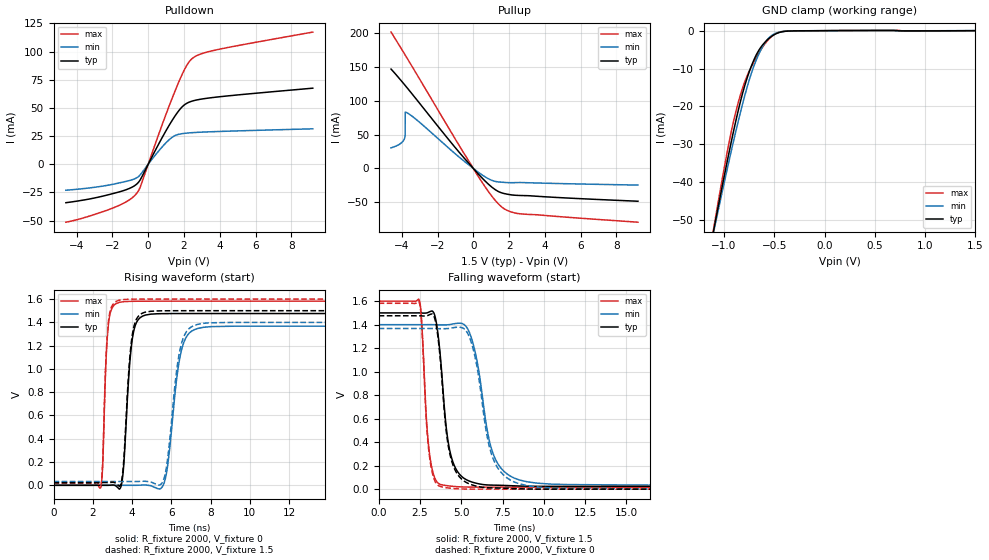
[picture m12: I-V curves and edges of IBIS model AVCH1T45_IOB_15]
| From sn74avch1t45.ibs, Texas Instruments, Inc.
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[Model]   AVCH1T45_IOB_15
Model_type  I/O
Vinl=0.49
Vinh=1.04
Enable   Active-High
Vref =   0
Rref =   2000
Cref =   15p
Vmeas =   0.75
| variable   typ   min   max
C_comp   5.30pF   4.64pF   5.89pF
| C_pullup   5.23pF   3.72pF   7.65pF
| C_pulldown   4.92pF   4.34pF   5.58pF
| C_tri-state   5.30pF   4.64pF   5.89pF
[Temperature Range]   40   100   -40
| Ambient temperature   25   85   -40
[Voltage range]   1.5   1.4   1.6
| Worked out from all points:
|   slope of the pulldown table from 0 to 0.225 V, typ, clamps not added: 32.1 ohm
|   slope of the pullup table from 0 to 0.225 V, typ, clamps not added: 33.9 ohm
|   GND clamp passes 1 mA (typ) near -0.50 V on its own axis
|   rising waveform, R_fixture 2000, V_fixture 0: 20-80 % time 334ps typ, 544ps min, 203ps max; typ from 0 V to 1.48 V
|   falling waveform, R_fixture 2000, V_fixture 1.5: 20-80 % time 639ps typ, 1.02ns min, 392ps max; typ from 1.5 V to 0.023 V
|   rising waveform, R_fixture 2000, V_fixture 1.5: 20-80 % time 330ps typ, 532ps min, 201ps max; typ from 0.023 V to 1.5 V
|   falling waveform, R_fixture 2000, V_fixture 0: 20-80 % time 639ps typ, 1.01ns min, 386ps max; typ from 1.48 V to 0 V
[GND Clamp]
| AVCH1T45_IOB_15
|   Voltage   I(typ)   I(min)   I(max)
-4.6V     -599.6mA   -548.2mA   -664.6mA
-1.1V     -52.36mA   -52.8mA    -51.85mA
-1.075V   -48.9mA    -49.67mA   -47.95mA
-930mV    -29.68mA   -32.07mA   -27.01mA
-880mV    -23.6mA    -26.34mA   -21.2mA
-830mV    -18.08mA   -20.9mA    -16.41mA
-765mV    -12.13mA   -14.48mA   -11.64mA
-685mV    -6.738mA   -8.147mA   -7.41mA
-605mV    -3.434mA   -3.729mA   -3.946mA
-535mV    -1.679mA   -1.475mA   -1.741mA
-370mV    -121.9uA   -99.54uA   -128.4uA
1.5V      812pA      11.73uA    -26.87uA
[Pulldown]
| AVCH1T45_IOB_15
|   Voltage   I(typ)   I(min)   I(max)
-4.6V     -34.07mA   -23.01mA   -51.35mA
-1.88V    -25.6mA    -17.43mA   -38.2mA
-1.09V    -21.68mA   -14.59mA   -31.97mA
-630mV    -17.39mA   -11.88mA   -25.55mA
-415mV    -12.94mA   -8.777mA   -18.95mA
595mV     18.22mA    11.97mA    26.91mA
1.27V     37.14mA    23.08mA    55.77mA
1.7V      47.29mA    26.56mA    72.61mA
2.03V     52.78mA    27.45mA    84.03mA
2.5V      56.24mA    28.09mA    94.31mA
3.84V     59.63mA    29.04mA    101.6mA
9.2V      67.51mA    31.46mA    117.2mA
[Pullup]
| AVCH1T45_IOB_15
|   Voltage   I(typ)   I(min)   I(max)
-4.6V     146.8mA    30.47mA    201.5mA
-4.1V     131.8mA    36.24mA    180.2mA
-3.85V    123.9mA    43.97mA    169.4mA
-3.81V    122.6mA    49.37mA    167.6mA
-3.805V   122.5mA    83.3mA     167.4mA
-3.785V   121.8mA    83.17mA    166.5mA
-3.155V   101.3mA    71.56mA    138.9mA
175mV     -5.197mA   -3.574mA   -7.497mA
980mV     -26.35mA   -16.94mA   -39.04mA
1.625V    -36.35mA   -20.39mA   -57.65mA
2.595V    -39.89mA   -20.78mA   -66.9mA
9.2V      -48.41mA   -24.54mA   -79.36mA
[Ramp]
| AVCH1T45_IOB_15
| variable   typ   min   max
dV/dt_r   0.91/3.44E-10   0.84/5.58E-10   0.96/2.08E-10
dV/dt_f   0.90/6.47E-10   0.83/1.02E-09   0.96/3.97E-10
R_load = 2000
[Rising Waveform]
| AVCH1T45_IOB_15
R_fixture =   2000
C_fixture =   0
L_fixture =   0
V_fixture =   0
V_fixture_min = 0
V_fixture_max = 0
|   Time   V(typ)   V(min)   V(max)
0s        19.41nV    97.7nV     527.1pV
2.425ns   23.61uV    1.698uV    -13.52mV
2.78ns    -69.49uV   -12.2uV    1.359V
3.32ns    -28.02mV   12.31uV    1.57V
4.015ns   1.261V     -139.9uV   1.581V
4.675ns   1.462V     2.678mV    1.582V
5.64ns    1.475V     25.06mV    1.582V
6.48ns    1.476V     1.136V     1.582V
7.37ns    1.476V     1.349V     1.582V
34.99ns   1.476V     1.367V     1.582V
[Falling Waveform]
| AVCH1T45_IOB_15
R_fixture =   2000
C_fixture =   0
L_fixture =   0
V_fixture =   1.5
V_fixture_min = 1.4
V_fixture_max = 1.6
|   Time   V(typ)   V(min)   V(max)
0s        1.5V       1.4V       1.6V
2.465ns   1.5V       1.4V       1.605V
3.06ns    1.508V     1.4V       323.4mV
3.765ns   1.083V     1.398V     39.43mV
4.185ns   423.8mV    1.399V     29.13mV
4.745ns   155.9mV    1.411V     21.27mV
5.705ns   58.29mV    1.245V     17.53mV
6.975ns   34.14mV    284.9mV    17.14mV
8.5ns     27.07mV    79.24mV    17.11mV
34.99ns   23.4mV     32.34mV    17.1mV
[Rising Waveform]
| AVCH1T45_IOB_15
R_fixture =   2000
C_fixture =   0
L_fixture =   0
V_fixture =   1.5
V_fixture_min = 1.4
V_fixture_max = 1.6
|   Time   V(typ)   V(min)   V(max)
0s        23.4mV     32.34mV    17.1mV
2.425ns   23.42mV    32.34mV    4.291mV
2.775ns   23.31mV    32.32mV    1.375V
3.325ns   -5.038mV   32.35mV    1.589V
4.005ns   1.286V     32.2mV     1.599V
4.64ns    1.486V     34.87mV    1.6V
5.62ns    1.499V     55.27mV    1.6V
6.44ns    1.5V       1.165V     1.6V
7.32ns    1.5V       1.382V     1.6V
34.99ns   1.5V       1.4V       1.6V
[Falling Waveform]
| AVCH1T45_IOB_15
R_fixture =   2000
C_fixture =   0
L_fixture =   0
V_fixture =   0
V_fixture_min = 0
V_fixture_max = 0
|   Time   V(typ)   V(min)   V(max)
0s        1.476V     1.367V     1.582V
2.465ns   1.476V     1.367V     1.586V
3.035ns   1.482V     1.367V     328mV
3.735ns   1.099V     1.366V     23.05mV
4.17ns    409.2mV    1.367V     11.32mV
4.73ns    136mV      1.378V     3.697mV
5.685ns   34.98mV    1.213V     376.9uV
6.93ns    10.72mV    259.5mV    38.8uV
8.49ns    3.323mV    46.84mV    7.899uV
34.99ns   65.4nV     1.638uV    58.19nV
